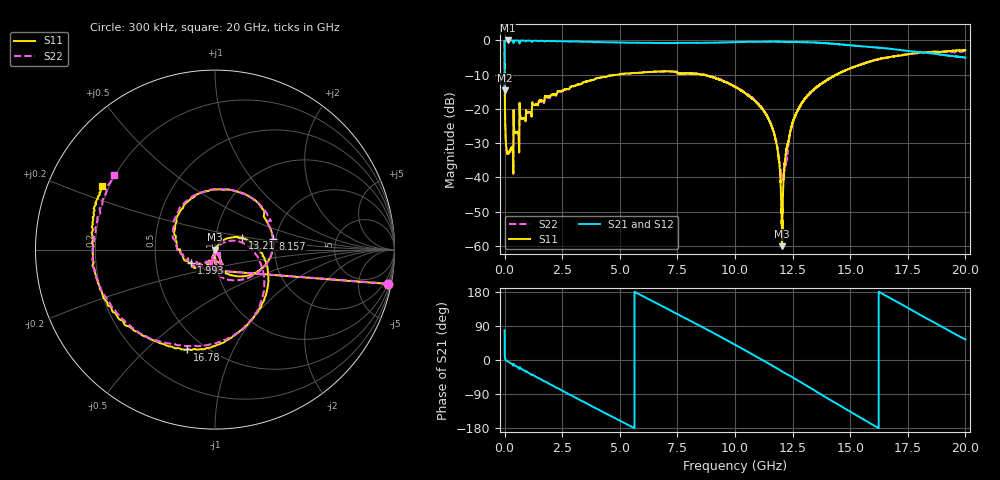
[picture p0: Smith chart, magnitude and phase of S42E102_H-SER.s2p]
!{S42E102}
!Johanson Technology Inc.
!www.johansontechnology.com
!Test Board Conditions:
!Substrate Type  RO4350B
!Substrate Thickness  50 mil
!Substrate Dk  3.66
!TL Type: GCPW
!TL Trace Width  60 mil
!TL Gap  10 mil
!Electrode orientation  Horizontal
!DUT TOPOLOGY	SERIES
!Mounting Pad LxW  14x55 mil
! Created Wed Nov 25 21:54:22 2020
# khz S ma R 50
! 2 Port Network Data from SP1.SP block
! freq  magS11  angS11  magS21  angS21  magS12  angS12  magS22  angS22
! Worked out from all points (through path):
!   20001 points, 300 kHz to 20 GHz, reference 50 ohm
!   highest |S21| = 0.00 dB at 145.3 MHz (marker M1); lowest = -14.5 dB at 300 kHz (marker M2)
!   group delay of S21, straight-line fit = 92.9 ps
!   lowest |S11| = -60.1 dB at 12.04 GHz (marker M3), VSWR 1.00, Z = 49.9 - j0.0219 ohm
!   |S11| at or under -10 dB: 4.714 MHz to 4.943 GHz (4.938 GHz wide, 200 % of centre); 8.595 GHz to 14.39 GHz (5.791 GHz wide, 50.4 % of centre); 14.38864 GHz to 14.39825 GHz (9.609 MHz wide, 0.0668 % of centre)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
!   |S22| runs from -40.7 to -0.2 dB; largest |S21 - S12| = 0.019
!   S11 on the Smith chart (normalised r, x): 300 kHz: 1, -10; 1.993 GHz: 0.76, -0.11; 8.157 GHz: 1.93, +0.26; 13.21 GHz: 1.35, +0.18; 16.78 GHz: 0.40, -0.68; 20 GHz: 0.17, +0.26
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300  0.9799 -11.2  0.1881 78.2  0.1884 79.1  0.982 -11.1
103300  0.02341 -91.9  0.9993 -2.6  0.9985 -2.6  0.02306 -92.4
145300  0.02204 -94.5  0.9997 -4.3  0.9989 -4.2  0.02208 -95.3
741300  0.07198 -114.0  0.9947 -23.8  0.9959 -23.8  0.07066 -113.7
1993300  0.1527 -151.2  0.9762 -64.8  0.9764 -64.8  0.1485 -155.0
3334300  0.2317 160.7  0.9565 -107.7  0.9566 -107.8  0.2314 166.4
5120300  0.3252 105.4  0.9329 -163.7  0.9316 -163.7  0.3246 109.2
6667300  0.3509 60.2  0.9201 147.5  0.9174 147.5  0.351 56.8
8157300  0.3278 10.4  0.9232 100.2  0.9169 100.4  0.328 10.2
1.00003e7  0.2097 -45.3  0.9435 40.3  0.9455 40.4  0.2127 -53.2
1.15073e7  0.06551 -93.1  0.9607 -11.1  0.9617 -11.0  0.06601 -103.9
1.18193e7  0.02874 -104.8  0.9591 -22.1  0.9608 -22.0  0.03017 -104.8
1.20373e7  0.0009867 -167.1  0.9567 -30.0  0.9582 -30.0  0.01011 -51.9
1.22283e7  0.02506 53.4  0.9489 -36.6  0.9489 -36.8  0.01718 27.1
1.24723e7  0.05825 51.9  0.9446 -44.6  0.9476 -44.9  0.05727 39.0
1.32113e7  0.1654 23.0  0.937 -71.5  0.9379 -71.5  0.1609 12.8
1.33343e7  0.1812 18.3  0.9353 -76.0  0.9348 -75.8  0.178 7.9
1.51693e7  0.4105 -52.0  0.8371 -141.9  0.8448 -142.5  0.4148 -55.1
1.66673e7  0.5691 -102.2  0.7615 165.9  0.7477 165.8  0.5635 -107.9
1.67803e7  0.578 -105.7  0.7566 161.9  0.7399 161.9  0.5732 -111.8
1.83273e7  0.6772 -160.8  0.6568 109.4  0.6588 110.2  0.668 -159.2
2e7  0.7244 150.5  0.5604 54.4  0.5625 55.4  0.6974 143.6
